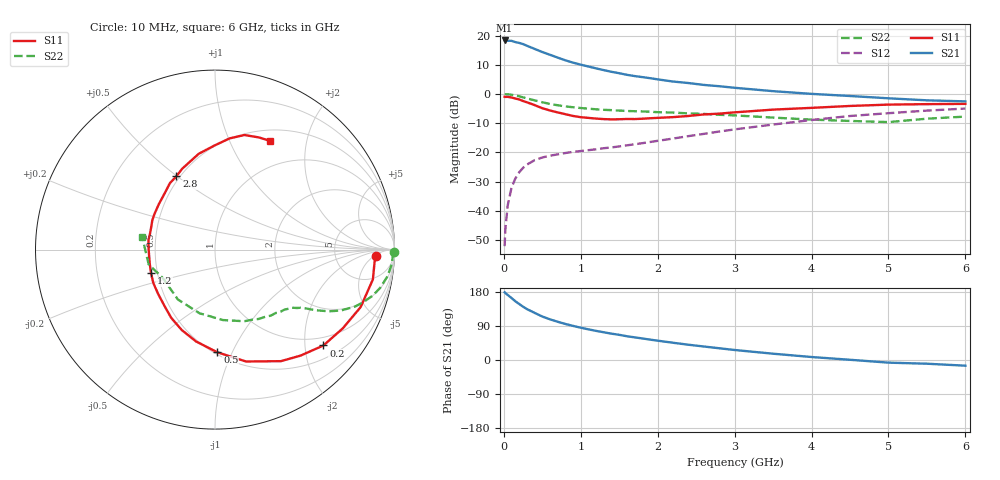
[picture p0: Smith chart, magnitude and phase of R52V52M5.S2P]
! SIEMENS Small Signal Semiconductors
! BFR183
! Si NPN RF Bipolar Junction Transistor in SOT23
! VCE = 2.5 V  IC = 2.5 mA
! Common Emitter S-Parameters:  May  1996
# GHz  S  MA  R  50
!  f  S11  S21  S12  S22
! GHz  MAG  ANG  MAG  ANG  MAG  ANG  MAG  ANG
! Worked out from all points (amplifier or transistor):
!   36 points, 10 MHz to 6 GHz, reference 50 ohm
!   highest |S21| = 18.3 dB at 10 MHz (marker M1)
!   |S21| within 3 dB of that: start of sweep to 410.4 MHz
!   unconditionally stable (mu >= 1): 1.303 GHz to 2.78 GHz
!   at 250 MHz: K = 0.27, MSG = 21.2 dB, |S12| = -25.2 dB
!   at 1.4 GHz: K = 1.04, MAG = 11.8 dB, |S12| = -18.3 dB
!   at 6 GHz: K = 0.90, MSG = 1.2 dB, |S12| = -5.0 dB
!   S11 on the Smith chart (normalised r, x): 10 MHz: 16, -6; 200 MHz: 0.79, -2.42; 500 MHz: 0.52, -0.88; 1.2 GHz: 0.46, -0.14; 2.8 GHz: 0.48, +0.50; 6 GHz: 0.63, +1.42
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0.01  0.8972 -2.2  8.242 178.6  0.0025 93.0  0.996 -0.9
0.02  0.8918 -4.3  8.149 176.6  0.0049 91.1  0.9906 -1.9
0.05  0.8952 -10.7  8.156 171.7  0.0124 85.7  0.9892 -4.5
0.1  0.8725 -21.5  8.116 163.5  0.0251 78.8  0.9723 -8.8
0.15  0.8366 -31.6  7.723 155.0  0.036 72.5  0.945 -13.0
0.2  0.8063 -41.5  7.475 147.7  0.0459 67.8  0.9153 -16.3
0.25  0.759 -51.1  7.145 140.6  0.0547 63.6  0.8767 -19.5
0.3  0.7221 -59.4  6.692 134.4  0.062 59.9  0.8416 -22.2
0.4  0.647 -74.5  5.91 124.4  0.0739 54.3  0.7796 -25.8
0.5  0.5722 -88.7  5.223 114.7  0.0822 50.7  0.7229 -28.4
0.6  0.5224 -101.7  4.687 107.3  0.0882 48.0  0.6755 -30.2
0.7  0.4851 -112.4  4.196 100.9  0.0929 46.5  0.6422 -31.5
0.8  0.4517 -122.7  3.771 95.1  0.098 45.5  0.614 -32.5
1.1  0.3908 -151.5  2.953 80.9  0.1096 46.0  0.5615 -35.4
1.2  0.3799 -159.8  2.745 76.8  0.1135 47.0  0.548 -36.3
1.6  0.3744 172.0  2.13 62.7  0.1325 50.2  0.5129 -40.6
2.2  0.4025 141.0  1.634 45.5  0.1731 53.9  0.4816 -49.8
2.8  0.4618 117.7  1.36 31.0  0.2283 53.4  0.4412 -62.4
3.5  0.5412 99.7  1.119 16.6  0.3006 48.4  0.3951 -83.5
4.5  0.625 82.5  0.925 0.6  0.4209 36.5  0.3464 -126.7
5.5  0.6712 68.6  0.78 -9.8  0.5205 22.6  0.3786 -167.4
6  0.6786 63.4  0.748 -15.0  0.5641 13.6  0.4112 170.2
